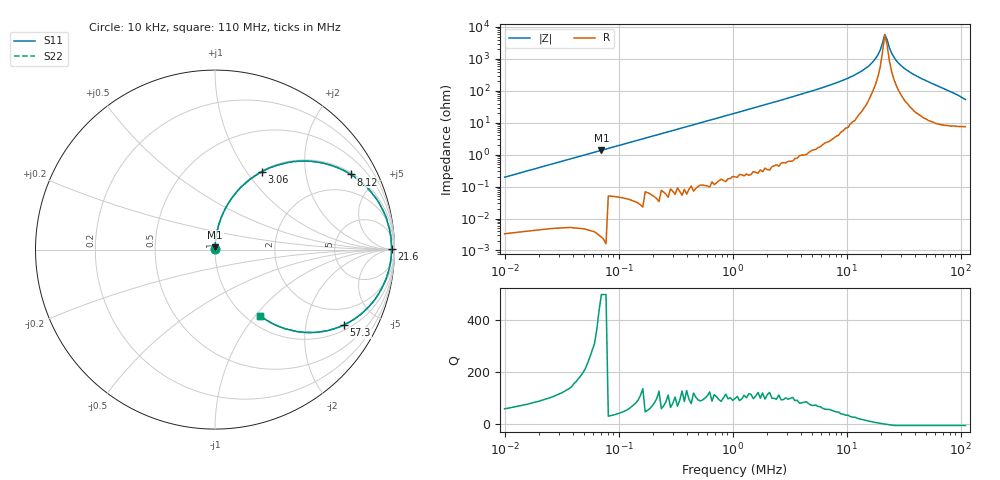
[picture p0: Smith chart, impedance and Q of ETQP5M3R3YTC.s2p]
! *** S-Parameter ***
!Copyright (C)  Panasonic Industry Corporation
!Power Inductors for Automotive application
!Parts No. ETQP5M3R3YTC
# HZ S RI R 50.000000
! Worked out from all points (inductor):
!   201 points, 10 kHz to 110 MHz, reference 50 ohm
!   read as one part in series: L = 3.13 uH near 10.5 kHz
!   highest Q = 531 at 70.6 kHz (marker M1), where L = 3.09 uH
!   self-resonance near 21.6 MHz
!   S11 on the Smith chart (normalised r, x): 10 kHz: 1.00, +0.00; 3.06 MHz: 1.01, +1.18; 8.12 MHz: 1.08, +3.56; 21.6 MHz: open; 57.3 MHz: 1.21, -3.29; 110 MHz: 1.15, -1.06
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10000  7.43e-05 0.00197  1 -0.00197  1 -0.00197  7.43e-05 0.00197
48600  0.000275 0.00947  1 -0.00947  1 -0.00947  0.000275 0.00947
70600  0.000427 0.0137  1 -0.0137  1 -0.0137  0.000427 0.0137
226000  0.00242 0.0432  0.998 -0.0432  0.998 -0.0432  0.00242 0.0432
1050000  0.04 0.191  0.96 -0.191  0.96 -0.191  0.04 0.191
1830000  0.111 0.31  0.889 -0.31  0.889 -0.31  0.111 0.31
3060000  0.261 0.434  0.739 -0.434  0.739 -0.434  0.261 0.434
5100000  0.51 0.493  0.49 -0.493  0.49 -0.493  0.51 0.493
8120000  0.756 0.419  0.244 -0.419  0.244 -0.419  0.756 0.419
1.13e7  0.885 0.301  0.115 -0.301  0.115 -0.301  0.885 0.301
1.56e7  0.96 0.158  0.0401 -0.158  0.0401 -0.158  0.96 0.158
1.88e7  0.98 0.0707  0.0203 -0.0707  0.0203 -0.0707  0.98 0.0707
1.97e7  0.982 0.0487  0.0179 -0.0487  0.0179 -0.0487  0.982 0.0487
2.16e7  0.984 0.00472  0.0162 -0.00472  0.0162 -0.00472  0.984 0.00472
2.26e7  0.983 -0.0173  0.0168 0.0173  0.0168 0.0173  0.983 -0.0173
2.37e7  0.982 -0.0393  0.0184 0.0393  0.0184 0.0393  0.982 -0.0393
2.6e7  0.975 -0.0834  0.0247 0.0834  0.0247 0.0834  0.975 -0.0834
3.13e7  0.95 -0.171  0.0503 0.171  0.0503 0.171  0.95 -0.171
3.95e7  0.891 -0.278  0.109 0.278  0.109 0.278  0.891 -0.278
5.73e7  0.719 -0.419  0.281 0.419  0.281 0.419  0.719 -0.419
7.94e7  0.494 -0.461  0.506 0.461  0.506 0.461  0.494 -0.461
1.1e8  0.252 -0.369  0.748 0.369  0.748 0.369  0.252 -0.369
